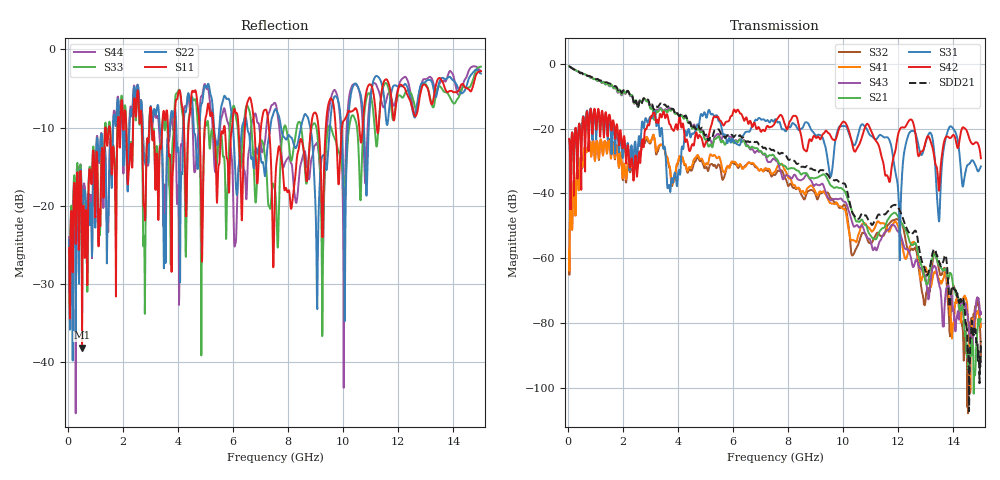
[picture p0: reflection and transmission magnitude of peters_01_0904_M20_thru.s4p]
# MHZ S RI R 50.00
! FREQ  S11  S12  S13  S14
!  S21  S22  S23  S24
!  S31  S32  S33  S34
!  S41  S42  S43  S44
!  REAL  IMAG  REAL  IMAG  REAL  IMAG  REAL  IMAG
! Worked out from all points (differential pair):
!   1496 points, 50 MHz to 15 GHz, reference 50 ohm
!   strongest paths, dB at 50 MHz, 3.79 GHz, 7.53 GHz, 11.27 GHz, 15 GHz:
!     S42: -23.1, -20.1, -18.0, -24.8, -29.1
!     S31: -23.2, -35.5, -17.1, -22.5, -31.6
!     S21: -0.7, -14.1, -28.9, -52.5, -78.8
!     S43: -0.6, -13.9, -29.7, -56.3, -77.3
!     S41: -57.6, -37.1, -33.2, -48.6, -81.3
!     S32: -58.5, -37.6, -34.3, -52.2, -90.2
!   taken as a pair (ports 1,3 in; 2,4 out), SDD21 dB: -0.6, -13.8, -27.2, -46.6, -85.7
!   lowest |S11| = -38.2 dB at 520 MHz (marker M1), VSWR 1.02, Z = 49 - j0.662 ohm
!   |S11| at or under -10 dB: start of sweep to 1.368 GHz; 3.053 GHz to 3.428 GHz (374.3 MHz wide, 11.6 % of centre); 7.303 GHz to 8.832 GHz (1.529 GHz wide, 19 % of centre)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
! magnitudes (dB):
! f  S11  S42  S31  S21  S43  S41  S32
! 50 MHz  -25.4  -23.1  -23.2  -0.7  -0.6  -57.6  -58.5
! 520 MHz  -38.2  -20.6  -19.7  -2.8  -2.8  -31.4  -31.7
! 3.13 GHz  -10.7  -15.0  -14.7  -17.1  -16.0  -22.2  -22.5
! 3.68 GHz  -13.7  -18.2  -37.4  -14.1  -13.4  -31.2  -31.8
! 7.75 GHz  -14.0  -15.8  -19.6  -30.9  -33.8  -30.9  -32.9
! 12.05 GHz  -4.6  -20.3  -57.7  -48.1  -52.1  -51.7  -48.5
! 15 GHz  -2.8  -29.1  -31.6  -78.8  -77.3  -81.3  -90.2
